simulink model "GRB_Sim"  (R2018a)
settings: Solver=ode4  StartTime=0.0  StopTime=12000  FixedStep=Ts  MaxStep=0.000001  RelTol=1e-12  AbsTol=1e-8  EnableMultiTasking=on
InitFcn:
  | start
StopFcn:
  | pl
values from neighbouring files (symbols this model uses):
  Cw2b = [ 0,          0,          0    [start.m]    (also in run.m)
  d2r = pi/180    (= 0.0174532925199)    [start.m]    (also in run.m; runf.m; orbitic.m; Quan.m)
  Hmax = 10    [start.m]    (also in run.m)
  Jw = [Iw, 0, 0    [start.m]    (also in run.m)
  Kq1 = I22*ww^2 - 3*wo2*(I11-I33)    [start.m]    (also in run.m)
  Kq2 = 2*I22*zet*ww    [start.m]    (also in run.m)
  Kqi = 0.0005    [start.m]    (also in run.m)
  Kr1 = (0.1*I11*I33*zet^2/Hy0) - sqrt( ((0.01^zet^4*I11^2*I33^2)/Hy0^2)+(4*I11*I33*zet^2) )    [start.m]    (also in run.m)
  Kr2 = 0.05*Kr1    [start.m]    (also in run.m)
  Kr3 = 0.04*zet*(Kr2-Hy0) * sqrt(abs(Hy0/(I11*I33)))    [start.m]    (also in run.m)
  nt = 7    [start.m]    (also in run.m; runf.m)
  Tmax = 0.05    [start.m]    (also in run.m)
  Ts = 0.01    [start.m]    (also in run.m = 0.001; runf.m = 0.0005)
  Tsr = 0.01    [start.m]
  wo = 0.00113    [start.m]    (also in run.m)
undefined symbols (not defined in the file or in its folder): Agr, Bgr, Cgr, den, Dgr, DiscIntNeverNeededParam, dsen, nsen, num, Phase_Plane, RW_Steering
libraries: simulink x5

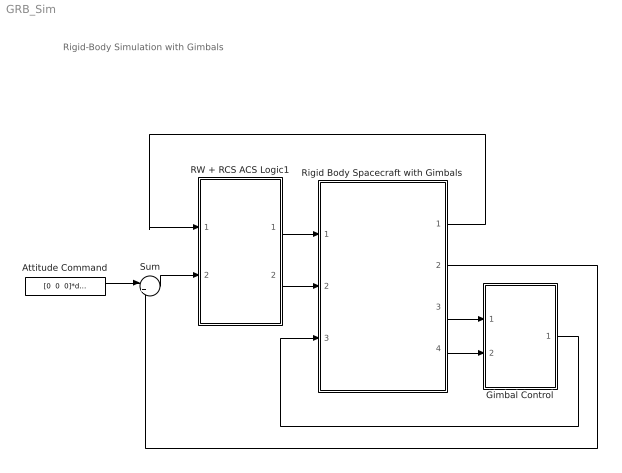
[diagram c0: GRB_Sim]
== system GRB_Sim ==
  note: Rigid-Body Simulation with Gimbals
  Attitude Command : Constant  Value="[0  0  0]*d2r"
  Gimbal Control : Subsystem
  RW + RCS ACS Logic1 : Subsystem
  Rigid Body Spacecraft with Gimbals : Subsystem
  Sum : Sum  Inputs=|+-
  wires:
  Attitude Command/1 -> Sum/1
  Sum/1 -> RW + RCS ACS Logic1/2(atter)
  Rigid Body Spacecraft with Gimbals/2(atti) -> Sum/2
  Rigid Body Spacecraft with Gimbals/1(Wr) -> RW + RCS ACS Logic1/1(wr(i))
  RW + RCS ACS Logic1/2(Trwi) -> Rigid Body Spacecraft with Gimbals/2(Trw(i))
  Gimbal Control/1(GTrq) -> Rigid Body Spacecraft with Gimbals/3(Tgimb)
  Rigid Body Spacecraft with Gimbals/3(alfa) -> Gimbal Control/1(Gimb)
  Rigid Body Spacecraft with Gimbals/4(alfad) -> Gimbal Control/2(Grate)
  RW + RCS ACS Logic1/1(Frcs) -> Rigid Body Spacecraft with Gimbals/1(Jet-7)

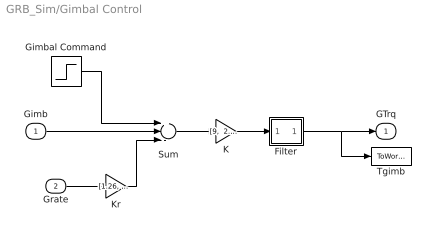
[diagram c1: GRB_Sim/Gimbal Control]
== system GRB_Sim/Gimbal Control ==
  Gimb : Inport
  Grate : Inport  Port=2
  Filter : Subsystem
  Gimbal Command : Step  After=[5, 5]*d2r  SampleTime=0
  K : Gain  Gain="[9,  2.85]"
  Kr : Gain  Gain="[1.26,  1.14]"
  Sum : Sum  Inputs=+--
  Tgimb : ToWorkspace  VariableName=Tgimb  SampleTime=-1
  GTrq : Outport
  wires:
  Sum/1 -> K/1
  Gimb/1 -> Sum/2
  Grate/1 -> Kr/1
  K/1 -> Filter/1(I)
  Kr/1 -> Sum/3
  Gimbal Command/1 -> Sum/1
  Filter/1(O) -> GTrq/1, Tgimb/1

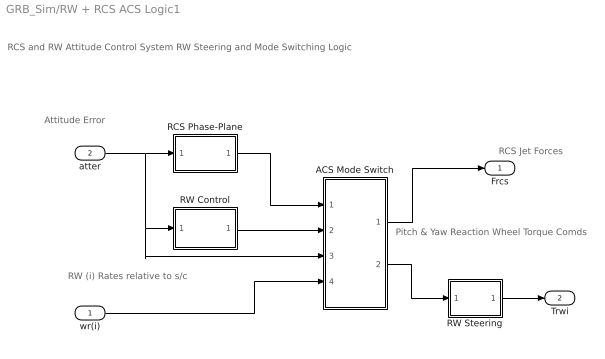
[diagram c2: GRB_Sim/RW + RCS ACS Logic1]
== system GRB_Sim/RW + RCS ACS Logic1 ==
  note: RCS and RW Attitude Control System RW Steering and Mode Switching Logic
  note: RCS Jet Forces
  note: RW (i) Rates relative to s/c
  note: Attitude Error
  note: Pitch & Yaw Reaction Wheel Torque Comds
  wr(i) : Inport
  atter : Inport  Port=2
  ACS Mode Switch : Subsystem
  RCS Phase-Plane : Subsystem
  RW Control : Subsystem
  RW Steering : Subsystem
  Frcs : Outport
  Trwi : Outport  Port=2
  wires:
  atter/1 -> ACS Mode Switch/3(atter), RW Control/1(atti), RCS Phase-Plane/1(atter)
  wr(i)/1 -> ACS Mode Switch/4(wr(i))
  RCS Phase-Plane/1(f(nt)) -> ACS Mode Switch/1(Frcs)
  RW Steering/1(Twi) -> Trwi/1
  ACS Mode Switch/1(" Frcs") -> Frcs/1
  ACS Mode Switch/2(" Trw") -> RW Steering/1(Trwc)
  RW Control/1(Tc) -> ACS Mode Switch/2(Trw)

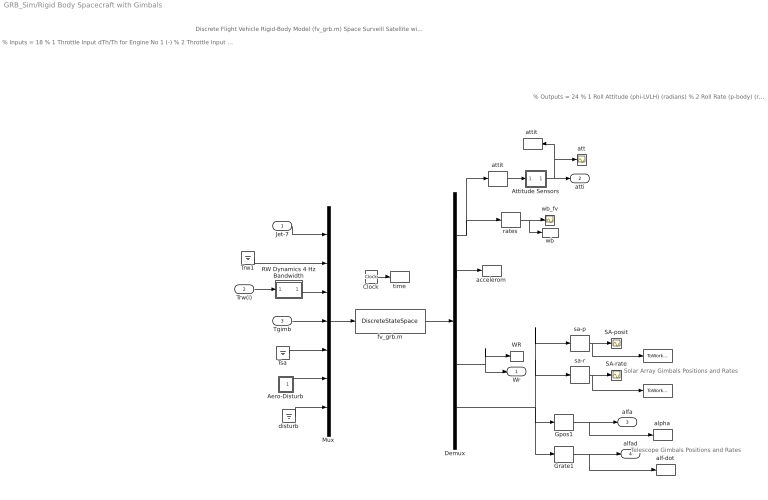
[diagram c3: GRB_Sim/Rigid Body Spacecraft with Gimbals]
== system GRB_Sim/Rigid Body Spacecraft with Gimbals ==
  note: % Inputs = 18 % 1 Throttle Input dTh/Th for Engine No 1 (-) % 2 Throttle Input dTh/Th for Engine No 2 (-) % 3 Throttle Input dTh/Th for Engine No 3 (-) % 4 Throttle Input dTh/Th for Engine No 4 (-) % 5 Throttle Input dTh/Th for Engine No 5 (-) % 6 Throttle Input dTh/Th for Engine No 6 (-) % 7 Throttle Input dTh/Th for Engine No 7 (-) % 8 Reaction Wheel No 1 Input Torque (ft-lb) % 9 Reaction Wheel No 2 Input Torque (ft-lb) % 10 Reaction Wheel No 3 Input Torque (ft-lb) % 11 Gimbaling Appendage Hinge # 1 Torque (ft-lb) % 12 Gimbaling Appendage Hinge # 2 Torque (ft-lb) % 13 Gimbaling Appendage Hinge # 3 Torque (ft-lb) % 14 Gimbaling Appendage Hinge # 4 Torque (ft-lb) % 15 External Torque Input 1 (ft-lb), direct: % 16 External Torque Input 2 (ft-lb), direct: % 17 External Torque Input 3 (ft-lb), direct: % 18 Ext Torque Direct.=( 0.1970 -0.5964 -0.7782)
  note: % Outputs = 24 % 1 Roll Attitude (phi-LVLH) (radians) % 2 Roll Rate (p-body) (rad/sec) % 3 Pitch Attitude (thet-LVLH) (radians) % 4 Pitch Rate (q-body) (rad/sec) % 5 Yaw Attitude (psi-LVLH) (radians) % 6 Yaw Rate (r-body) (rad/sec) % 7 Angle of attack, alfa, (radians) % 8 Angle of sideslip, beta, (radian) % 9 Change in Altitude, delta-h, (feet) % 10 Forward Acceleration (V-dot) (ft/sec) % 11 Cross Range Velocity (Vcr) (ft/sec) % 12 Accelerom # 1, (along X), (ft/sec^2) Translat. Acceler % 13 Accelerom # 2, (along Y), (ft/sec^2) Translat. Acceler % 14 Reaction Wheel # 1 Rate (rpm) relative to vehicle % 15 Reaction Wheel # 2 Rate (rpm) relative to vehicle % 16 Reaction Wheel # 3 Rate (rpm) relative to vehicle % 17 Gimbaling Appendage # 1 Relative Rotation, alfar( 1), % 18 Gimbaling Appendage # 1 Relative Rot.Rate, alfar-dot( % 19 Gimbaling Appendage # 2 Relative Rotation, alfar( 2), % 20 Gimbaling Appendage # 2 Relative Rot.Rate, alfar-dot( % 21 Gimbaling Appendage # 3 Relative Rotation, alfar( 3), % 22 Gimbaling Appendage # 3 Relative Rot.Rate, alfar-dot( % 23 Gimbaling Appendage # 4 Relative Rotation, alfar( 4), % 24 Gimbaling Appendage # 4 Relative Rot.Rate, alfar-dot(
  note: Discrete Flight Vehicle Rigid-Body Model (fv_grb.m) Space Surveill Satellite with RCS and Reaction Wheels (Gimbals, No Flex, Z-Transf)
  note: Telescope Gimbals Positions and Rates
  note: Solar Array Gimbals Positions and Rates
  Jet-7 : Inport
  Trw(i) : Inport  Port=2
  Tgimb : Inport  Port=3
  " " : ToWorkspace  VariableName=SA_pos  SampleTime=-1
  "   " : ToWorkspace  VariableName=SA_rate  SampleTime=-1
  Aero-Disturb : Subsystem
  Attitude Sensors : Subsystem
  Clock : Clock
  Demux : Demux  Outputs=[11, 2, 1,2, 8]
  Gpos1 : Selector  InputPortWidth=8  IndexOptions=Index vector (dialog)  Indices=[1,3]  OutputSizes=1
  Grate1 : Selector  InputPortWidth=8  IndexOptions=Index vector (dialog)  Indices=[2, 4]  OutputSizes=1
  Mux : Mux  Inputs=[7, 1,2, 2,2, 3,1]
  RW Dynamics 4 Hz Bandwidth : Subsystem
  SA-posit : Scope
  SA-rate : Scope
  Trw1 : Ground
  Tsa : Ground
  WR : ToWorkspace  VariableName=wr  SampleTime=-1
  accelerom : ToWorkspace  VariableName=accel  SampleTime=-1
  alf-dot : ToWorkspace  VariableName=alfad  SampleTime=-1
  alpha : ToWorkspace  VariableName=alfa  SampleTime=-1
  att : Scope
  attit : Selector  InputPortWidth=11  IndexOptions=Index vector (dialog)  Indices=[1, 3, 5]  OutputSizes=1
  "attit " : ToWorkspace  VariableName=atti  SampleTime=-1
  disturb : Ground
  fv_grb.m : DiscreteStateSpace  A=Agr  B=Bgr  C=Cgr  D=Dgr  SampleTime=Tsr
  rates : Selector  InputPortWidth=11  IndexOptions=Index vector (dialog)  Indices=[2, 4, 6]  OutputSizes=1
  sa-p : Selector  InputPortWidth=8  IndexOptions=Index vector (dialog)  Indices=[5, 7]  OutputSizes=1
  sa-r : Selector  InputPortWidth=8  IndexOptions=Index vector (dialog)  Indices=[6, 8]  OutputSizes=1
  time : ToWorkspace  VariableName=time  SampleTime=-1
  wb : ToWorkspace  VariableName=wb  SampleTime=-1
  wb_fv : Scope
  Wr : Outport
  atti : Outport  Port=2
  alfa : Outport  Port=3
  alfad : Outport  Port=4
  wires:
  Demux/4 -> Wr/1, WR/1
  Demux/1 -> rates/1, attit/1
  rates/1 -> wb_fv/1, wb/1
  attit/1 -> Attitude Sensors/1(I)
  Demux/2 -> accelerom/1
  Jet-7/1 -> Mux/1
  Trw(i)/1 -> RW Dynamics 4 Hz Bandwidth/1(I)
  Tgimb/1 -> Mux/4
  Aero-Disturb/1(Td) -> Mux/6
  disturb/1 -> Mux/7
  Tsa/1 -> Mux/5
  fv_grb.m/1 -> Demux/1
  Mux/1 -> fv_grb.m/1
  Trw1/1 -> Mux/2
  Attitude Sensors/1(O) -> atti/1, att/1, "attit "/1
  RW Dynamics 4 Hz Bandwidth/1(O) -> Mux/3
  Clock/1 -> time/1
  Demux/5 -> Gpos1/1, Grate1/1, sa-p/1, sa-r/1
  Grate1/1 -> alfad/1, alf-dot/1
  Gpos1/1 -> alfa/1, alpha/1
  sa-p/1 -> SA-posit/1, " "/1
  sa-r/1 -> SA-rate/1, "   "/1

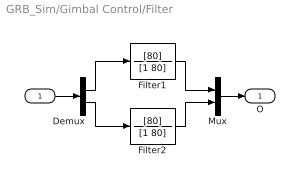
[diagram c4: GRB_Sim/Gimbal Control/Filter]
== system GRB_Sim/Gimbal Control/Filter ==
  I : Inport
  Demux : Demux  Outputs=2
  Filter1 : TransferFcn  Numerator=[80]  Denominator=[1 80]
  Filter2 : TransferFcn  Numerator=[80]  Denominator=[1 80]
  Mux : Mux  Inputs=2
  O : Outport
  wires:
  Mux/1 -> O/1
  I/1 -> Demux/1
  Demux/2 -> Filter2/1
  Demux/1 -> Filter1/1
  Filter2/1 -> Mux/2
  Filter1/1 -> Mux/1

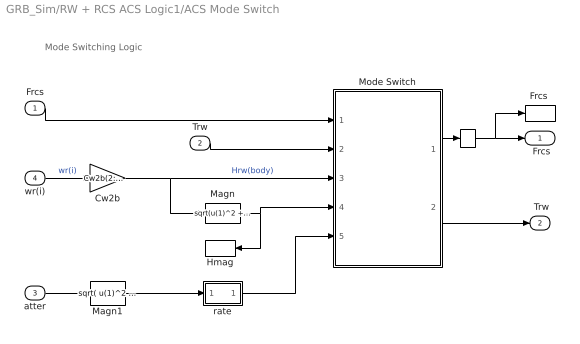
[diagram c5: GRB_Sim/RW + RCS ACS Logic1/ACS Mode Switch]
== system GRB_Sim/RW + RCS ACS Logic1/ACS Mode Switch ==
  note: Mode Switching Logic
  Frcs : Inport
  Trw : Inport  Port=2
  atter : Inport  Port=3
  wr(i) : Inport  Port=4
  "   " : Memory
  Cw2b : Gain  Gain=Cw2b(2:3,2:3)*Jw(2:3,2:3)  Multiplication=Matrix(K*u)
  "Frcs " : ToWorkspace  VariableName=Frcs  SampleTime=-1
  Hmag : ToWorkspace  VariableName=Hmag  SampleTime=-1
  Magn : Fcn  Expr=sqrt(u(1)^2 + u(2)^2)
  Magn1 : Fcn  Expr=sqrt( u(1)^2 + u(2)^2 + u(3)^2 )
  Mode Switch : Stateflow chart  TreatAsAtomicUnit=on
  rate : Subsystem
  " Frcs" : Outport
  " Trw" : Outport  Port=2
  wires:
  wr(i)/1 -> Cw2b/1  "wr(i)"
  Frcs/1 -> Mode Switch/1(Fi)
  Trw/1 -> Mode Switch/2(Tci)
  atter/1 -> Magn1/1
  Magn/1 -> Mode Switch/4(hmag), Hmag/1
  Mode Switch/1(Fo) -> "   "/1
  Mode Switch/2(Tco) -> " Trw"/1
  Cw2b/1 -> Mode Switch/3(hrwa), Magn/1  "Hrw(body)"
  Magn1/1 -> rate/1(in)
  rate/1(ou) -> Mode Switch/5(atter)
  "   "/1 -> "Frcs "/1, " Frcs"/1

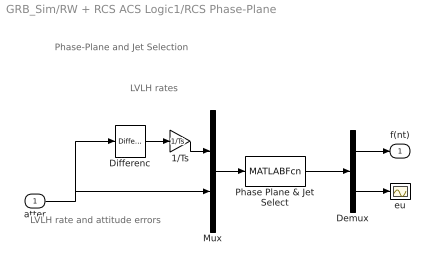
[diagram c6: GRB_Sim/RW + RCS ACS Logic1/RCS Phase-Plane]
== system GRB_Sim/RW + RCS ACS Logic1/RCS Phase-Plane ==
  note: Phase-Plane and Jet Selection
  note: LVLH rate and attitude errors
  note: LVLH rates
  atter : Inport
  1/Ts : Gain  Gain=1/Ts
  Demux : Demux  Outputs=[nt, 3]
  Differenc : simulink/Discrete/Difference  ICPrevInput=0.0  InputProcessing=Inherited  OutMin=[]  OutMax=[]  OutDataType=sfix(16)  OutScaling=2^-10  DoSatur=off
  Mux : Mux  Inputs="[3  3]"
  Phase Plane & Jet Select : MATLABFcn  MATLABFcn=Phase_Plane( u(1:3), u(4:6) )  OutputDimensions=nt + 3
  eu : Scope
  f(nt) : Outport
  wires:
  atter/1 -> Mux/2, Differenc/1
  1/Ts/1 -> Mux/1
  Demux/2 -> eu/1
  Demux/1 -> f(nt)/1
  Phase Plane & Jet Select/1 -> Demux/1
  Mux/1 -> Phase Plane & Jet Select/1
  Differenc/1 -> 1/Ts/1

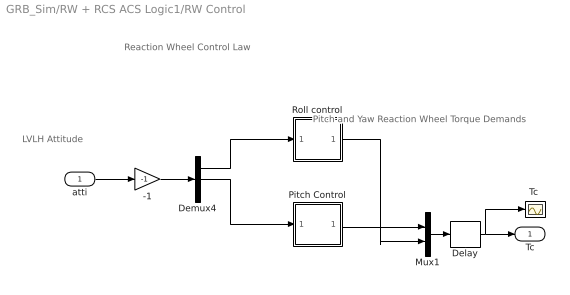
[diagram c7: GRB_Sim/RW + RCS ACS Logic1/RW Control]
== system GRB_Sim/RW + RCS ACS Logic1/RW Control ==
  note: Reaction Wheel Control Law
  note: LVLH Attitude
  note: Pitch and Yaw Reaction Wheel Torque Demands
  atti : Inport
  -1 : Gain  Gain=-1
  Delay : Delay  DelayLength=1  InputProcessing=Inherited  SampleTime=Tsr
  Demux4 : Demux  Outputs=3
  Mux1 : Mux  Inputs=2
  Pitch Control : Subsystem
  Roll control : Subsystem
  "Tc " : Scope
  Tc : Outport
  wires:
  Roll control/1(Tcz) -> Mux1/2
  -1/1 -> Demux4/1
  Mux1/1 -> Delay/1
  atti/1 -> -1/1
  Demux4/2 -> Pitch Control/1(the)
  Pitch Control/1(Tcy) -> Mux1/1
  Demux4/1 -> Roll control/1(phi)
  Delay/1 -> Tc/1, "Tc "/1

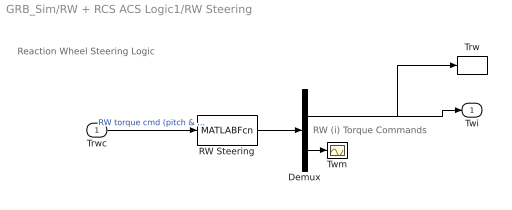
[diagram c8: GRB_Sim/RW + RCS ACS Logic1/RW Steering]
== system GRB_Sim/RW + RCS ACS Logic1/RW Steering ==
  note: RW (i) Torque Commands
  note: Reaction Wheel Steering Logic
  Trwc : Inport
  Demux : Demux  Outputs=[2, 1]
  RW Steering : MATLABFcn  MATLABFcn=RW_Steering( u(1:2) )  OutputDimensions=3
  Trw : ToWorkspace  VariableName=Trw  SampleTime=-1
  Twm : Scope
  Twi : Outport
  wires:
  Demux/2 -> Twm/1
  Demux/1 -> Trw/1, Twi/1
  RW Steering/1 -> Demux/1
  Trwc/1 -> RW Steering/1  "RW torque cmd (pitch & yaw)"

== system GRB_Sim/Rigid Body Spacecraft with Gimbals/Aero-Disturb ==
  note: Aerodynamic Disturbance Torques
  30 : Gain  Gain=5
  Disturb Trq1 : Sin  Amplitude="[0.0,   1,   0.2]*0.0001"  Bias="[0.0,  0.5,  0.15]*0.0001"  Frequency=[wo, wo, wo]  SampleTime=0
  Disturb Trq2 : Sin  Amplitude=[0, 1.2, 1]*0.0001  Bias=[0 0 0]  Frequency=[wo, wo, wo]*2  SampleTime=0
  Sum2 : Sum  Inputs=+|+
  "Td " : ToWorkspace  VariableName=Td  SampleTime=-1
  Td : Outport
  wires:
  30/1 -> "Td "/1, Td/1
  Disturb Trq2/1 -> Sum2/2  "2*wo"
  Sum2/1 -> 30/1
  Disturb Trq1/1 -> Sum2/1  "wo"

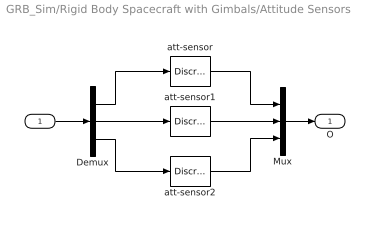
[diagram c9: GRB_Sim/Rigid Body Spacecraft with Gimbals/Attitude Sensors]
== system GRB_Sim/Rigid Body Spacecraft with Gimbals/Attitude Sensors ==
  I : Inport
  Demux : Demux  Outputs=3
  Mux : Mux  Inputs=3
  att-sensor : DiscreteTransferFcn  Numerator=[nsen]  Denominator=[dsen]  SampleTime=Ts
  att-sensor1 : DiscreteTransferFcn  Numerator=[nsen]  Denominator=[dsen]  SampleTime=Ts
  att-sensor2 : DiscreteTransferFcn  Numerator=[nsen]  Denominator=[dsen]  SampleTime=Ts
  O : Outport
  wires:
  I/1 -> Demux/1
  Mux/1 -> O/1
  att-sensor/1 -> Mux/1
  Demux/1 -> att-sensor/1
  Demux/3 -> att-sensor2/1
  att-sensor2/1 -> Mux/3
  Demux/2 -> att-sensor1/1
  att-sensor1/1 -> Mux/2

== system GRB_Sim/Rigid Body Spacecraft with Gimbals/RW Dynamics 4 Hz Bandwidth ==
  I : Inport
  Demux : Demux  Outputs=2
  Mux : Mux  Inputs=2
  RW Dynamics : DiscreteTransferFcn  Numerator="[0  0.221199217]"  Denominator=[1 -0.778800783]  SampleTime=Ts
  RW Dynamics1 : DiscreteTransferFcn  Numerator="[0  0.221199217]"  Denominator=[1 -0.778800783]  SampleTime=Ts
  O : Outport
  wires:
  Demux/2 -> RW Dynamics1/1
  Demux/1 -> RW Dynamics/1
  I/1 -> Demux/1
  Mux/1 -> O/1
  RW Dynamics/1 -> Mux/1
  RW Dynamics1/1 -> Mux/2

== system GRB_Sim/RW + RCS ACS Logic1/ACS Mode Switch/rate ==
  in : Inport
  1/Ts : Gain  Gain=1/Ts
  Abs : Abs
  Differenc : simulink/Discrete/Difference  ICPrevInput=0.0  InputProcessing=Inherited  OutMin=[]  OutMax=[]  OutDataType=sfix(16)  OutScaling=2^-10  DoSatur=off
  ou : Outport
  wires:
  Differenc/1 -> 1/Ts/1
  1/Ts/1 -> Abs/1
  in/1 -> Differenc/1
  Abs/1 -> ou/1

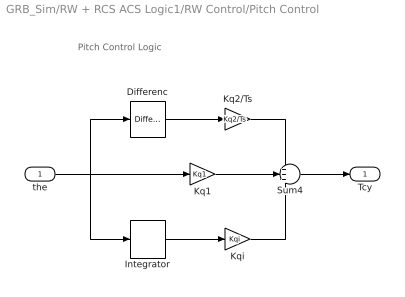
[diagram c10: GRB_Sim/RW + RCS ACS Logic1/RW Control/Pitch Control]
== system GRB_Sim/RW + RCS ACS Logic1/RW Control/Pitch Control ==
  note: Pitch Control Logic
  the : Inport
  Differenc : simulink/Discrete/Difference  ICPrevInput=0.0  InputProcessing=Inherited  OutMin=[]  OutMax=[]  OutDataType=sfix(16)  OutScaling=2^-10  DoSatur=off
  Integrator : DiscreteIntegrator  SampleTime=Ts  ICPrevOutput=DiscIntNeverNeededParam  ICPrevScaledInput=DiscIntNeverNeededParam
  Kq1 : Gain  Gain=Kq1
  Kq2/Ts : Gain  Gain=Kq2/Ts
  Kqi : Gain  Gain=Kqi
  Sum4 : Sum  Inputs=+++
  Tcy : Outport
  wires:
  Differenc/1 -> Kq2/Ts/1
  Integrator/1 -> Kqi/1
  Kqi/1 -> Sum4/3
  the/1 -> Differenc/1, Integrator/1, Kq1/1
  Kq2/Ts/1 -> Sum4/1
  Sum4/1 -> Tcy/1
  Kq1/1 -> Sum4/2

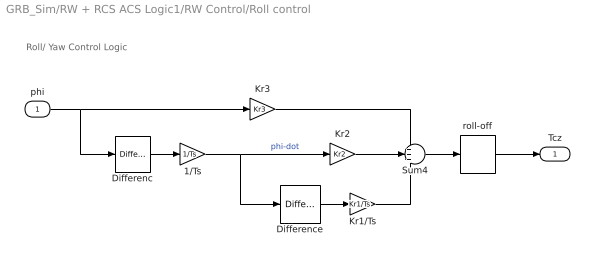
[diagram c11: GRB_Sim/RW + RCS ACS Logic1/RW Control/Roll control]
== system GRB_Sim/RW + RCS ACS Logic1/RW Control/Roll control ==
  note: Roll/ Yaw Control Logic
  phi : Inport
  1/Ts : Gain  Gain=1/Ts
  Differenc : simulink/Discrete/Difference  ICPrevInput=0.0  InputProcessing=Inherited  OutMin=[]  OutMax=[]  OutDataType=sfix(16)  OutScaling=2^-10  DoSatur=off
  Difference : simulink/Discrete/Difference  ICPrevInput=0.0  InputProcessing=Inherited  OutMin=[]  OutMax=[]  OutDataType=sfix(16)  OutScaling=2^-10  DoSatur=off
  Kr1/Ts : Gain  Gain=Kr1/Ts
  Kr2 : Gain  Gain=Kr2
  Kr3 : Gain  Gain=Kr3
  Sum4 : Sum  Inputs=+++
  roll-off : DiscreteTransferFcn  Numerator=[num]  Denominator=[den]  SampleTime=Ts
  Tcz : Outport
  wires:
  1/Ts/1 -> Difference/1, Kr2/1  "phi-dot"
  Differenc/1 -> 1/Ts/1
  Difference/1 -> Kr1/Ts/1
  Sum4/1 -> roll-off/1
  phi/1 -> Differenc/1, Kr3/1
  Kr1/Ts/1 -> Sum4/3
  Kr2/1 -> Sum4/2
  Kr3/1 -> Sum4/1
  roll-off/1 -> Tcz/1

== stateflow chart GRB_Sim/RW + RCS
ACS Logic1/ACS Mode 
Switch/Mode Switch ==
  state RCS1
    en:Fo=Fi;
    en:Tco=-hrwa*Tmax/hmag;
  state RCS2
    en:Fo=Fi;
    en:Tco=Tz;
  state RW
    en:Fo=Fz;
    en:Tco=Tci;
  RCS2 -> RCS1 : [hmag>Hmax/10]
  RCS1 -> RCS1 : [hmag>=Hmax/10 ... || atter>=Rlim]
  RCS1 -> (junction 13)
  (junction 13) -> RCS2
  (junction 13) -> RW : [hmag<Hmax/10 ... && atter<Rlim]
  RW -> RCS1 : [hmag>=Hmax]
  RCS2 -> RW : [atter<Rlim]
  (default) -> RW
  RW -> RW : [hmag<Hmax]
  data: Fi input; Tci input; Fo output double; Tco output double; Tmax parameter double; Hmax parameter double; hrwa input; hmag input; Fz constant double; atter input; Tz constant double; Rlim constant double =0.8e-3
